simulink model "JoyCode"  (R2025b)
settings: Solver=FixedStepAuto  StartTime=0.0  StopTime=inf  RelTol=1e-3
libraries: arduinolib x13

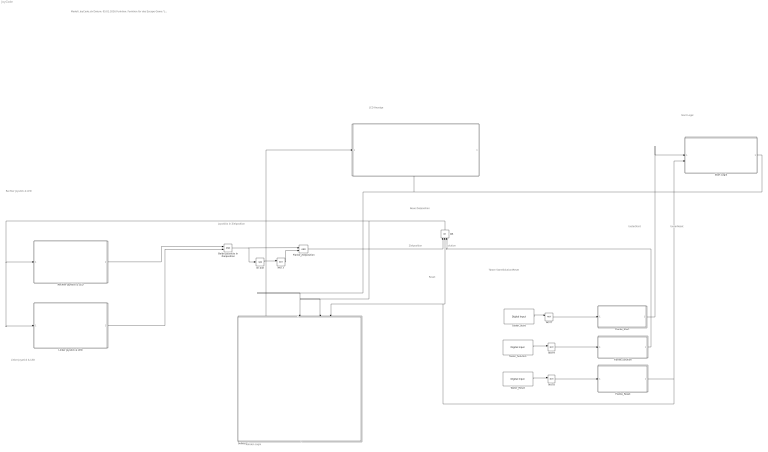
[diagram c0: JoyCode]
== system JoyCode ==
  note: Modell: JoyCode.slx Datum: 05.01.2026 Funktion: Funktion für das Escape-Game "JoyCode". Die Logik ist in mehreren Subsysteme unterteilt Implementierung: Simulink 2025b Autor: Jens Potthoff, Mohammed Yassine Houari
  note: Solution
  note: Reset
  note: Zielposition
  note: tasterStart
  note: tasterReset
  note: Neue Zielposition
  note: Taster Start/Solution/Reset
  note: Start Logik
  note: LCD Anzeige
  note: Linker Joystick & LED
  note: Rechter Joystick & LED
  note: Joysticks in Zielposition
  note: Runden Logik
  " " : Subsystem
  Beide Joysticks in Zielposition : Logic  IconShape=distinctive  AllPortsSameDT=off  OutDataTypeStr=boolean
  Flanke_Reset : Subsystem
  Flanke_Solution : Subsystem
  Flanke_Start : Subsystem
  Flanke_Zielposition : Logic  IconShape=distinctive  AllPortsSameDT=off  OutDataTypeStr=boolean
  Im Ziel : UnitDelay  SampleTime=-1  HasFrameUpgradeWarning=on
  Linker Joystick & LED : Subsystem
  NOT{3,7..9} (4 alike) : Logic  Operator=NOT  IconShape=distinctive  AllPortsSameDT=off  OutDataTypeStr=boolean
  OR : Logic  Operator=OR  Inputs=3  IconShape=distinctive  AllPortsSameDT=off  OutDataTypeStr=boolean
  Rechter Joystick & LED : Subsystem
  Start Logik : Subsystem
  Subsystem : Subsystem
  Taster_Reset : arduinolib/Digital Input  pinNumber=12  mode=Input Pullup  Direction=input  SampleTime=0.01  blockPlatform=arduino
  Taster_Solution : arduinolib/Digital Input  pinNumber=8  mode=Input Pullup  Direction=input  SampleTime=0.01  blockPlatform=arduino
  Taster_Start : arduinolib/Digital Input  pinNumber=13  mode=Input Pullup  Direction=input  SampleTime=0.01  blockPlatform=arduino
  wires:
  Im Ziel/1 -> NOT3/1
  NOT3/1 -> Flanke_Zielposition/2
  Flanke_Zielposition/1 -> OR/1
  Taster_Start/1 -> NOT7/1
  Taster_Solution/1 -> NOT9/1
  Taster_Reset/1 -> NOT8/1
  Beide Joysticks in Zielposition/1 -> Flanke_Zielposition/1, Im Ziel/1
  NOT7/1 -> Flanke_Start/1(In)
  NOT9/1 -> Flanke_Solution/1(In)
  Flanke_Reset/1(Out) -> Start Logik/2(tasterReset), Subsystem/3(In Reset), OR/2
  NOT8/1 -> Flanke_Reset/1(In)
  Flanke_Start/1(Out) -> Start Logik/1(tasterStart)
  OR/1 -> Subsystem/2(In Zielposition), Linker Joystick & LED/1(rundeGewechselt), Rechter Joystick & LED/1(rundeGewechselt)
  Flanke_Solution/1(Out) -> OR/3
  Start Logik/1(spielLaeuft_in) -> Subsystem/1(In Start), " "/2(spielLaeuft)
  Rechter Joystick & LED/1(Out) -> Beide Joysticks in Zielposition/1
  Linker Joystick & LED/1(Out) -> Beide Joysticks in Zielposition/2
  Subsystem/1(Out Setze Runde) -> " "/1(runde)

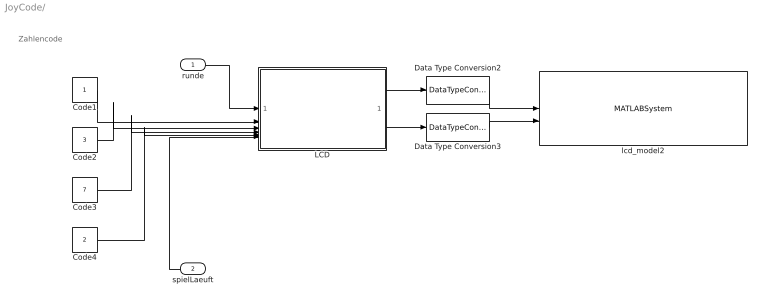
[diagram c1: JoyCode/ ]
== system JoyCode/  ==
  note: Zahlencode
  runde : Inport
  spielLaeuft : Inport  Port=2
  Code1 : Constant
  Code2 : Constant  Value=3
  Code3 : Constant  Value=7
  Code4 : Constant  Value=2
  Data Type Conversion2 : DataTypeConversion  OutDataTypeStr=uint8
  Data Type Conversion3 : DataTypeConversion  OutDataTypeStr=uint8
  LCD : MATLAB Function  TreatAsAtomicUnit=on
  lcd_model2 : MATLABSystem  System=lcd  SampleTime=-1
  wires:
  LCD/1(zeile1) -> Data Type Conversion2/1
  Data Type Conversion2/1 -> lcd_model2/1
  Code3/1 -> LCD/4(code3)
  Data Type Conversion3/1 -> lcd_model2/2
  runde/1 -> LCD/1(runde)
  LCD/2(zeile2) -> Data Type Conversion3/1
  Code4/1 -> LCD/5(code4)
  Code2/1 -> LCD/3(code2)
  Code1/1 -> LCD/2(code1)
  spielLaeuft/1 -> LCD/6(spielLaeuft)

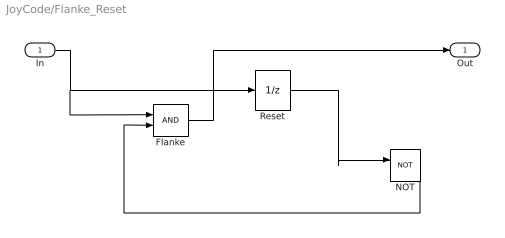
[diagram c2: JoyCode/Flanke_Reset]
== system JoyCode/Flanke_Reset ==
  In : Inport
  Flanke : Logic  IconShape=distinctive  AllPortsSameDT=off  OutDataTypeStr=boolean
  NOT : Logic  Operator=NOT  IconShape=distinctive  AllPortsSameDT=off  OutDataTypeStr=boolean
  Reset : UnitDelay  SampleTime=-1  HasFrameUpgradeWarning=on
  Out : Outport
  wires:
  In/1 -> Flanke/1, Reset/1
  Flanke/1 -> Out/1
  NOT/1 -> Flanke/2
  Reset/1 -> NOT/1

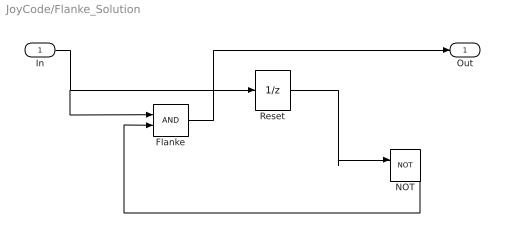
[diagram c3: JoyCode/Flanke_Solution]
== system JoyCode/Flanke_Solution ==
  In : Inport
  Flanke : Logic  IconShape=distinctive  AllPortsSameDT=off  OutDataTypeStr=boolean
  NOT : Logic  Operator=NOT  IconShape=distinctive  AllPortsSameDT=off  OutDataTypeStr=boolean
  Reset : UnitDelay  SampleTime=-1  HasFrameUpgradeWarning=on
  Out : Outport
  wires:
  In/1 -> Flanke/1, Reset/1
  Flanke/1 -> Out/1
  NOT/1 -> Flanke/2
  Reset/1 -> NOT/1

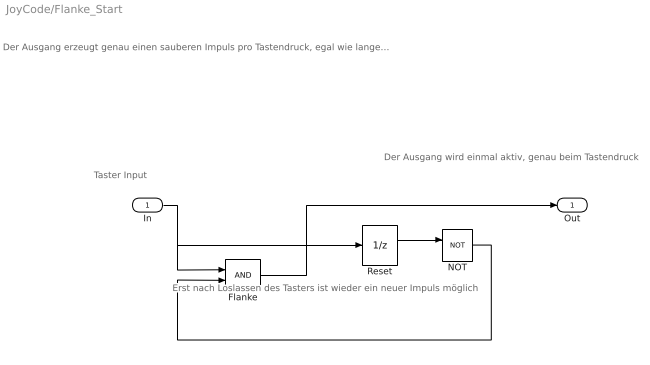
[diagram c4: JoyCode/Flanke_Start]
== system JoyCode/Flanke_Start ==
  note: Der Ausgang erzeugt genau einen sauberen Impuls pro Tastendruck, egal wie lange oder wie unruhig der Taster gedrückt wird. Vorteil: keine Mehrfachauslösung und kein Prellen.
  note: Der Ausgang wird einmal aktiv, genau beim Tastendruck
  note: Erst nach Loslassen des Tasters ist wieder ein neuer Impuls möglich
  note: Taster Input
  In : Inport
  Flanke : Logic  IconShape=distinctive  AllPortsSameDT=off  OutDataTypeStr=boolean
  NOT : Logic  Operator=NOT  IconShape=distinctive  AllPortsSameDT=off  OutDataTypeStr=boolean
  Reset : UnitDelay  SampleTime=-1  HasFrameUpgradeWarning=on
  Out : Outport
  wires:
  In/1 -> Flanke/1, Reset/1
  Flanke/1 -> Out/1
  NOT/1 -> Flanke/2
  Reset/1 -> NOT/1

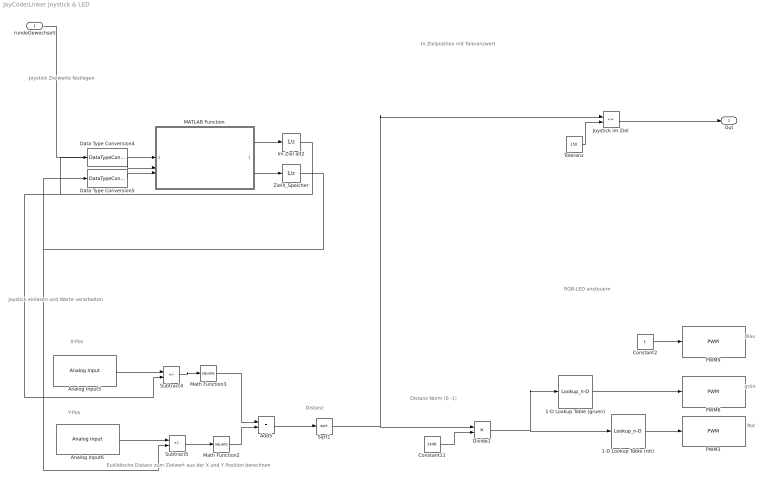
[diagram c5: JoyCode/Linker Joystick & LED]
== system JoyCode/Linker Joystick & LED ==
  note: Distanz
  note: Distanz Norm (0 -1)
  note: Rot
  note: Blau
  note: X-Pos
  note: grün
  note: RGB-LED ansteuern
  note: Y-Pos
  note: Joystick einlesen und Werte verarbeiten
  note: Joystick Zielwerte festlegen
  note: In Zielposition mit Toleranzwert
  note: Euklidische Distanz zum Zielwert aus der X und Y Position berechnen
  rundeGewechselt : Inport
  1-D Lookup Table (gruen) : Lookup_n-D  NumberOfTableDimensions=1  BreakpointsForDimension1=[0;0.10000000000000001;0.25;0.5;1]  Table=[80;50;20;0;0]  ExtrapMethod=Clip  InternalRulePriority=Speed  RndMeth=Simplest
  1-D Lookup Table (rot) : Lookup_n-D  NumberOfTableDimensions=1  BreakpointsForDimension1=[0;0.10000000000000001;0.25;0.5;1]  Table=[0;40;80;100;100]  ExtrapMethod=Clip  InternalRulePriority=Speed  RndMeth=Simplest
  Add5 : Sum
  Analog Input5 : arduinolib/Analog Input  pinNumber=0  ReadResultsOnly=off  ConversionTriggerSource=Software  ExternalTriggerType=uint32( 0 )  OutputDataType=uint16  EnableConversionCompleteNotify=off  EnableOuputStatus=off  SampleTime=0.01  blockPlatform=arduino
  Analog Input6 : arduinolib/Analog Input  pinNumber=1  ReadResultsOnly=off  ConversionTriggerSource=Software  ExternalTriggerType=uint32( 0 )  OutputDataType=uint16  EnableConversionCompleteNotify=off  EnableOuputStatus=off  SampleTime=0.01  blockPlatform=arduino
  Constant11 : Constant  Value=1448
  Constant2 : Constant
  Data Type Conversion4 : DataTypeConversion  OutDataTypeStr=double
  Data Type Conversion5 : DataTypeConversion  OutDataTypeStr=double
  Divide1 : Product  Inputs=*/
  Im Ziel alt2 : UnitDelay  InitialCondition=859  SampleTime=-1  HasFrameUpgradeWarning=on
  Joystick im Ziel : RelationalOperator  Operator=<=  OutDataTypeStr=boolean  RndMeth=Simplest
  MATLAB Function : MATLAB Function  TreatAsAtomicUnit=on
  Math Function2 : Math  Operator=square
  Math Function3 : Math  Operator=square
  PWM3 : arduinolib/PWM  pinNumber=9  frequencyType=Default  desiredFrequency=50  achievableFrequency=490.2
  PWM6 : arduinolib/PWM  pinNumber=11  frequencyType=Default  desiredFrequency=50  achievableFrequency=490.2
  PWM9 : arduinolib/PWM  pinNumber=10  frequencyType=Default  desiredFrequency=50  achievableFrequency=490.2
  Sqrt1 : Sqrt
  Subtract4 : Sum  Inputs=+-
  Subtract5 : Sum  Inputs=+-
  Toleranz : Constant  Value=150
  ZielX_Speicher : UnitDelay  InitialCondition=34  SampleTime=-1  HasFrameUpgradeWarning=on
  Out : Outport
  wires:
  Constant11/1 -> Divide1/2
  MATLAB Function/1(zielX_out) -> Im Ziel alt2/1
  Add5/1 -> Sqrt1/1
  Data Type Conversion4/1 -> MATLAB Function/2(zielX_in)
  Im Ziel alt2/1 -> Data Type Conversion4/1, Subtract4/2
  Constant2/1 -> PWM9/1
  Math Function2/1 -> Add5/2
  Math Function3/1 -> Add5/1
  Subtract4/1 -> Math Function3/1
  Data Type Conversion5/1 -> MATLAB Function/3(zielY_in)
  Sqrt1/1 -> Divide1/1, Joystick im Ziel/1
  Analog Input6/1 -> Subtract5/1
  Subtract5/1 -> Math Function2/1
  ZielX_Speicher/1 -> Data Type Conversion5/1, Subtract5/2
  Toleranz/1 -> Joystick im Ziel/2
  Analog Input5/1 -> Subtract4/1
  MATLAB Function/2(zielY_out) -> ZielX_Speicher/1
  rundeGewechselt/1 -> MATLAB Function/1(rundeGewechselt)
  Joystick im Ziel/1 -> Out/1
  Divide1/1 -> 1-D Lookup Table (rot)/1, 1-D Lookup Table (gruen)/1
  1-D Lookup Table (rot)/1 -> PWM3/1
  1-D Lookup Table (gruen)/1 -> PWM6/1

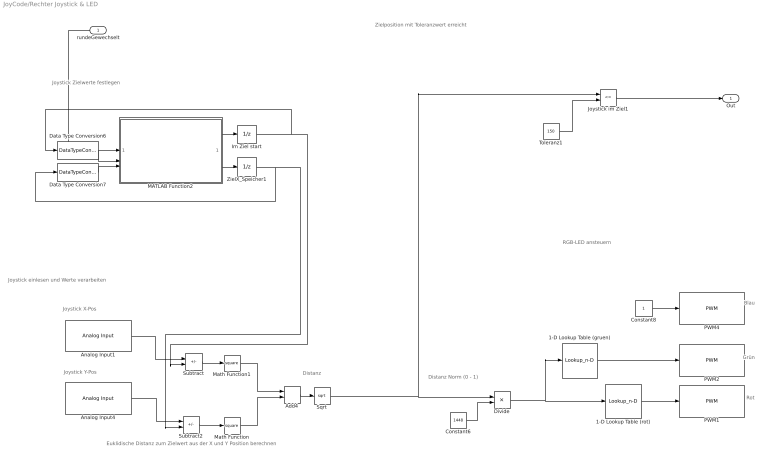
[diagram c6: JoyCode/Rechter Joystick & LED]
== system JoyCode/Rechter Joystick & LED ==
  note: Euklidische Distanz zum Zielwert aus der X und Y Position berechnen
  note: Zielposition mit Toleranzwert erreicht
  note: Joystick einlesen und Werte verarbeiten
  note: Blau
  note: Grün
  note: Rot
  note: Distanz
  note: Joystick X-Pos
  note: Distanz Norm (0 - 1)
  note: Joystick Y-Pos
  note: RGB-LED ansteuern
  note: Joystick Zielwerte festlegen
  rundeGewechselt : Inport
  1-D Lookup Table (gruen) : Lookup_n-D  NumberOfTableDimensions=1  BreakpointsForDimension1=[0;0.10000000000000001;0.25;0.5;1]  Table=[80;50;20;0;0]  ExtrapMethod=Clip  InternalRulePriority=Speed  RndMeth=Simplest
  1-D Lookup Table (rot) : Lookup_n-D  NumberOfTableDimensions=1  BreakpointsForDimension1=[0;0.10000000000000001;0.25;0.5;1]  Table=[0;40;80;100;100]  ExtrapMethod=Clip  InternalRulePriority=Speed  RndMeth=Simplest
  Add4 : Sum
  Analog Input1 : arduinolib/Analog Input  pinNumber=3  ReadResultsOnly=off  ConversionTriggerSource=Software  ExternalTriggerType=uint32( 0 )  OutputDataType=uint16  EnableConversionCompleteNotify=off  EnableOuputStatus=off  SampleTime=0.01  blockPlatform=arduino
  Analog Input4 : arduinolib/Analog Input  pinNumber=2  ReadResultsOnly=off  ConversionTriggerSource=Software  ExternalTriggerType=uint32( 0 )  OutputDataType=uint16  EnableConversionCompleteNotify=off  EnableOuputStatus=off  SampleTime=0.01  blockPlatform=arduino
  Constant6 : Constant  Value=1448
  Constant8 : Constant
  Data Type Conversion6 : DataTypeConversion  OutDataTypeStr=double
  Data Type Conversion7 : DataTypeConversion  OutDataTypeStr=double
  Divide : Product  Inputs=*/
  Im Ziel start : UnitDelay  InitialCondition=900  SampleTime=-1  HasFrameUpgradeWarning=on
  Joystick im Ziel1 : RelationalOperator  Operator=<=  OutDataTypeStr=boolean  RndMeth=Simplest
  MATLAB Function2 : MATLAB Function  TreatAsAtomicUnit=on
  Math Function : Math  Operator=square
  Math Function1 : Math  Operator=square
  PWM1 : arduinolib/PWM  pinNumber=5  frequencyType=Default  desiredFrequency=50  achievableFrequency=490.2
  PWM2 : arduinolib/PWM  pinNumber=3  frequencyType=Default  desiredFrequency=50  achievableFrequency=490.2
  PWM4 : arduinolib/PWM  pinNumber=6  frequencyType=Default  desiredFrequency=50  achievableFrequency=490.2
  Sqrt : Sqrt
  Subtract : Sum  Inputs=+-
  Subtract2 : Sum  Inputs=+-
  Toleranz1 : Constant  Value=150
  ZielX_Speicher1 : UnitDelay  InitialCondition=780  SampleTime=-1  HasFrameUpgradeWarning=on
  Out : Outport
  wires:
  Analog Input1/1 -> Subtract/1
  ZielX_Speicher1/1 -> Subtract2/2, Data Type Conversion7/1
  Constant6/1 -> Divide/2
  Analog Input4/1 -> Subtract2/1
  MATLAB Function2/1(zielX_out) -> Im Ziel start/1
  Subtract2/1 -> Math Function/1
  Divide/1 -> 1-D Lookup Table (rot)/1, 1-D Lookup Table (gruen)/1
  Data Type Conversion6/1 -> MATLAB Function2/2(zielX_in)
  Im Ziel start/1 -> Data Type Conversion6/1, Subtract/2
  Joystick im Ziel1/1 -> Out/1
  rundeGewechselt/1 -> MATLAB Function2/1(rundeGewechselt)
  Add4/1 -> Sqrt/1
  MATLAB Function2/2(zielY_out) -> ZielX_Speicher1/1
  Math Function/1 -> Add4/2
  Math Function1/1 -> Add4/1
  Data Type Conversion7/1 -> MATLAB Function2/3(zielY_in)
  Subtract/1 -> Math Function1/1
  Toleranz1/1 -> Joystick im Ziel1/2
  Constant8/1 -> PWM4/1
  Sqrt/1 -> Joystick im Ziel1/1, Divide/1
  1-D Lookup Table (rot)/1 -> PWM1/1
  1-D Lookup Table (gruen)/1 -> PWM2/1

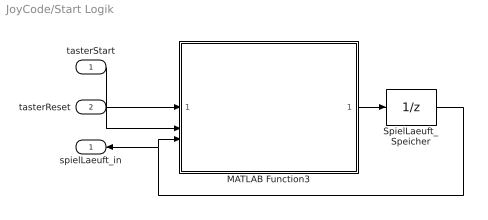
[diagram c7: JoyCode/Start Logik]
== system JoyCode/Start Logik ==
  tasterStart : Inport
  tasterReset : Inport  Port=2
  MATLAB Function3 : MATLAB Function  TreatAsAtomicUnit=on
  SpielLaeuft_Speicher : UnitDelay  SampleTime=-1  HasFrameUpgradeWarning=on
  spielLaeuft_in : Outport
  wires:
  tasterStart/1 -> MATLAB Function3/1(tasterStart)
  SpielLaeuft_Speicher/1 -> spielLaeuft_in/1, MATLAB Function3/3(spielLaeuft_in)
  MATLAB Function3/1(spielLaeuft_out) -> SpielLaeuft_Speicher/1
  tasterReset/1 -> MATLAB Function3/2(tasterReset)

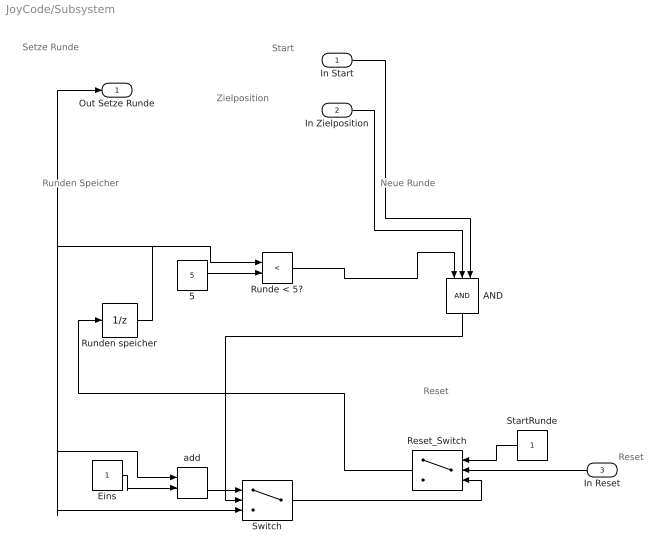
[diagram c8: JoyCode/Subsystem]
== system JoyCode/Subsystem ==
  note: Neue Runde
  note: Reset
  note: Runden Speicher
  note: Start
  note: Zielposition
  note: Reset
  note: Setze Runde
  In Start : Inport
  In Zielposition : Inport  Port=2
  In Reset : Inport  Port=3
  5 : Constant  Value=5
  AND : Logic  Inputs=3  IconShape=distinctive  AllPortsSameDT=off  OutDataTypeStr=boolean
  Eins : Constant
  Reset_Switch : Switch  Criteria=u2 ~= 0
  Runde < 5? : RelationalOperator  Operator=<  OutDataTypeStr=boolean  RndMeth=Simplest
  Runden speicher : UnitDelay  InitialCondition=1  SampleTime=-1  HasFrameUpgradeWarning=on
  StartRunde : Constant
  Switch : Switch  Criteria=u2 ~= 0
  add : Sum
  Out Setze Runde : Outport
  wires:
  Reset_Switch/1 -> Runden speicher/1
  Eins/1 -> add/2
  Switch/1 -> Reset_Switch/3
  AND/1 -> Switch/2
  Runden speicher/1 -> Out Setze Runde/1, Switch/3, add/1, Runde < 5?/1
  In Zielposition/1 -> AND/2
  5/1 -> Runde < 5?/2
  StartRunde/1 -> Reset_Switch/1
  add/1 -> Switch/1
  Runde < 5?/1 -> AND/1
  In Start/1 -> AND/3
  In Reset/1 -> Reset_Switch/2

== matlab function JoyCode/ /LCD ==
function [zeile1,zeile2]=LCD_Logik(runde,code1,code2,code3,code4,spielLaeuft)

zeile1=zeros(16,1);
zeile2=zeros(16,1);
rundeLCD = runde-1;
% WENN SPIEL NOCH NICHT GESTARTET
if spielLaeuft == 0
    % Obere Zeile: "Druecke START   "
    % D=68 r=114 u=117 e=101 c=99 k=107 e=101 Space=32 S=83 T=84 A=65 R=82 T=84
    zeile1(1)=68;   % D
    zeile1(2)=114;  % r
    zeile1(3)=117;  % u
    zeile1(4)=101;  % e
    zeile1(5)=99;   % c
    zeile1(6)=107;  % k
    zeile1(7)=101;  % e
    zeile1(8)=32;   % Space
    zeile1(9)=83;   % S
    zeile1(10)=84;  % T
    zeile1(11)=65;  % A
    zeile1(12)=82;  % R
    zeile1(13)=84;  % T
    zeile1(14)=32;  % Space
    zeile1(15)=32;  % Space
    zeile1(16)=32;  % Space
    
    % Untere Zeile: "um zu beginnen  "
    % u=117 m=109 Space=32 z=122 u=117 Space=32 b=98 e=101 g=103 i=105 n=110 n=110 e=101 n=110
    zeile2(1)=117;  % u
    zeile2(2)=109;  % m
    zeile2(3)=32;   % Space
    zeile2(4)=122;  % z
    zeile2(5)=117;  % u
    zeile2(6)=32;   % Space
    zeile2(7)=98;   % b
    zeile2(8)=101;  % e
    zeile2(9)=103;  % g
    zeile2(10)=105; % i
    zeile2(11)=110; % n
    zeile2(12)=110; % n
    zeile2(13)=101; % e
    zeile2(14)=110; % n
    zeile2(15)=32;  % Space
    zeile2(16)=32;  % Space
    
    return;
end

% AB HIER: SPIEL LÄUFT

freigeschaltet=runde-1;
if freigeschaltet>4
    freigeschaltet=4;
end
if freigeschaltet<0
    freigeschaltet=0;
end

% OBERE ZEILE
if runde>=5
    zeile1(1)=70;
    zeile1(2)=101;
    zeile1(3)=114;
    zeile1(4)=116;
    zeile1(5)=105;
    zeile1(6)=103;
    zeile1(7)=33;
    zeile1(8:16)=32;
else
    zeile1(1)=90;
    zeile1(2)=97;
    zeile1(3)=104;
    zeile1(4)=108;
    zeile1(5)=101;
    zeile1(6)=110;
    zeile1(7)=99;
    zeile1(8)=111;
    zeile1(9)=100;
    zeile1(10)=101;
    zeile1(11)=58;
    zeile1(12)=48+rundeLCD;
    zeile1(13)=47;
    zeile1(14)=52;
    zeile1(15)=32;
    zeile1(16)=32;
end

% UNTERE ZEILE
zeile2(:)=32;

if freigeschaltet>=1
    zeile2(1)=48+code1;
else
    zeile2(1)=45;
end

if freigeschaltet>=2
    zeile2(5)=48+code2;
else
    zeile2(5)=45;
end

if freigeschaltet>=3
    zeile2(9)=48+code3;
else
    zeile2(9)=45;
end

if freigeschaltet>=4
    zeile2(13)=48+code4;
else
    zeile2(13)=45;
end

end

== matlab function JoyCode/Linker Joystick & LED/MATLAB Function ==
function [zielX_out, zielY_out] = zielGenerator(rundeGewechselt, zielX_in, zielY_in)

%% ===== EINSTELLBARE PARAMETER =====

% Min- und Max-Werte
minVal = 30;
maxVal = 980;

% Ausschlusszone (Werte um die Mitte herum ausschließen)
ausschlussMitte  = 512;    % Zentrum der Ausschlusszone
ausschlussBreite = 20;     % +/- dieser Wert wird ausgeschlossen

% Ausschlusszone Grenzen
ausschlussMin = ausschlussMitte - ausschlussBreite;
ausschlussMax = ausschlussMitte + ausschlussBreite;

% Größe der Ausschlusszone
ausschlussGroesse = ausschlussMax - ausschlussMin + 1;

% Effektive Spannweite (ohne Ausschlusszone)
effektiveRange = (maxVal - minVal + 1) - ausschlussGroesse;

% Wenn die Runde gerade gewechselt hat, neue Position
if rundeGewechselt == 1
    
    % Temporäre Werte im effektiven Bereich berechnen
    tempX = mod(zielX_in * 7 + zielY_in * 3 + 137, effektiveRange);
    tempY = mod(zielY_in * 11 + zielX_in * 5 + 251, effektiveRange);
    
    % Auf gültige Bereiche mappen (Lücke überspringen)
    zielX_out = mappeAufGueltig(tempX, minVal, ausschlussMin, ausschlussMax);
    zielY_out = mappeAufGueltig(tempY, minVal, ausschlussMin, ausschlussMax);
    
else
    % Sonst: Werte beibehalten
    zielX_out = zielX_in;
    zielY_out = zielY_in;
end

end

%% ===== HILFSFUNKTION =====
function wert = mappeAufGueltig(temp, minVal, ausschlussMin, ausschlussMax)
    % Bereich 1: minVal bis (ausschlussMin - 1)
    bereich1Groesse = ausschlussMin - minVal;
    
    if temp < bereich1Groesse
        % Wert liegt im unteren gültigen Bereich
        wert = minVal + temp;
    else
        % Wert liegt im oberen gültigen Bereich (Lücke überspringen)
        wert = ausschlussMax + 1 + (temp - bereich1Groesse);
    end
end

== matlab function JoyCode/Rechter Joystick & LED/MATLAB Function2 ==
function [zielX_out, zielY_out] = zielGenerator(rundeGewechselt, zielX_in, zielY_in)

%% ===== EINSTELLBARE PARAMETER =====

% Min- und Max-Werte
minVal = 30;
maxVal = 980;

% Ausschlusszone (Werte um die Mitte herum ausschließen)
ausschlussMitte  = 512;    % Zentrum der Ausschlusszone
ausschlussBreite = 20;     % +/- dieser Wert wird ausgeschlossen

% Ausschlusszone Grenzen
ausschlussMin = ausschlussMitte - ausschlussBreite;
ausschlussMax = ausschlussMitte + ausschlussBreite;

% Größe der Ausschlusszone
ausschlussGroesse = ausschlussMax - ausschlussMin + 1;

% Effektive Spannweite (ohne Ausschlusszone)
effektiveRange = (maxVal - minVal + 1) - ausschlussGroesse;

% Wenn die Runde gerade gewechselt hat, neue Position
if rundeGewechselt == 1
    
    % Temporäre Werte im effektiven Bereich berechnen
    tempX = mod(zielX_in * 7 + zielY_in * 3 + 137, effektiveRange);
    tempY = mod(zielY_in * 11 + zielX_in * 5 + 251, effektiveRange);
    
    % Auf gültige Bereiche mappen (Lücke überspringen)
    zielX_out = mappeAufGueltig(tempX, minVal, ausschlussMin, ausschlussMax);
    zielY_out = mappeAufGueltig(tempY, minVal, ausschlussMin, ausschlussMax);
    
else
    % Sonst: Werte beibehalten
    zielX_out = zielX_in;
    zielY_out = zielY_in;
end

end

%% ===== HILFSFUNKTION =====
function wert = mappeAufGueltig(temp, minVal, ausschlussMin, ausschlussMax)
    % Bereich 1: minVal bis (ausschlussMin - 1)
    bereich1Groesse = ausschlussMin - minVal;
    
    if temp < bereich1Groesse
        % Wert liegt im unteren gültigen Bereich
        wert = minVal + temp;
    else
        % Wert liegt im oberen gültigen Bereich (Lücke überspringen)
        wert = ausschlussMax + 1 + (temp - bereich1Groesse);
    end
end

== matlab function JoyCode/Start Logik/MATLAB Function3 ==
function spielLaeuft_out = StartLogik(tasterStart, tasterReset, spielLaeuft_in)

% Standardmäßig bleibt der Zustand gleich
spielLaeuft_out = spielLaeuft_in;

% Wenn Reset gedrückt wird, Spiel stoppen
if tasterReset == 1
    spielLaeuft_out = 0;
end

% Wenn Start gedrückt wird UND Spiel noch nicht läuft, Spiel starten
if tasterStart == 1 && spielLaeuft_in == 0
    spielLaeuft_out = 1;
end

end
